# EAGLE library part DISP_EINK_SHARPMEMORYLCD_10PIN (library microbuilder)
Sharp Mono Memory LCD LS013B4DN02 - 1.35" 96x96 Pixels LS027B7DH01 - 2.7" 400x240 Pixels
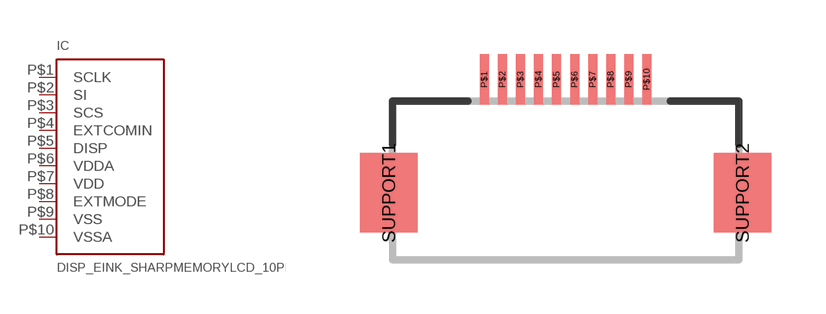
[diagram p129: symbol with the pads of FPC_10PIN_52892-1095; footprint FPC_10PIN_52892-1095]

Designator prefix IC

## DISP_EINK_SHARPMEMORYLCD_10PIN  [FPC_10PIN_52892-1095]
P$1  SCLK  in
P$2  SI  in
P$3  SCS  in
P$4  EXTCOMIN  in
P$5  DISP  in
P$6  VDDA  pwr
P$7  VDD  pwr
P$8  EXTMODE  in
P$9  VSS  pwr
P$10  VSSA  pwr

## Footprint FPC_10PIN_52892-1095 (pad centres in mm)
Source: http://www.molex.com/pdm_docs/sd/528921095_sd.pdf
smd 0.25 x 1.4: P$1 -2.25,0; P$2 -1.75,0; P$3 -1.25,0; P$4 -0.75,0; P$5 -0.25,0; P$6 0.25,0; P$7 0.75,0; P$8 1.25,0; P$9 1.75,0; P$10 2.25,0
smd 1.6 x 2.2: SUPPORT1 -4.9,-3.15; SUPPORT2 4.9,-3.15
